TYPE ST_EL5131_INPUT :
STRUCT
	{attribute 'displaymode':='bin'}
	Status							:	ST_Status_UDINT_TO_BIT;// Size=4.0
	Counter_value					:	UDINT;
	Latch_value						:	UDINT;
	Latch_value2					:	UDINT;
	{attribute 'displaymode':='bin'}
	Status_OutputChn1				:	ST_Status_OutputChn_UINT_TO_BIT;
	TimestampChn1					:	ARRAY[1..8] OF ULINT;
	
	{attribute 'displaymode':='bin'}
	Status_OutputChn2				:	ST_Status_OutputChn_UINT_TO_BIT;
	TimestampChn2					:	ARRAY[1..8] OF ULINT;
END_STRUCT
END_TYPE
